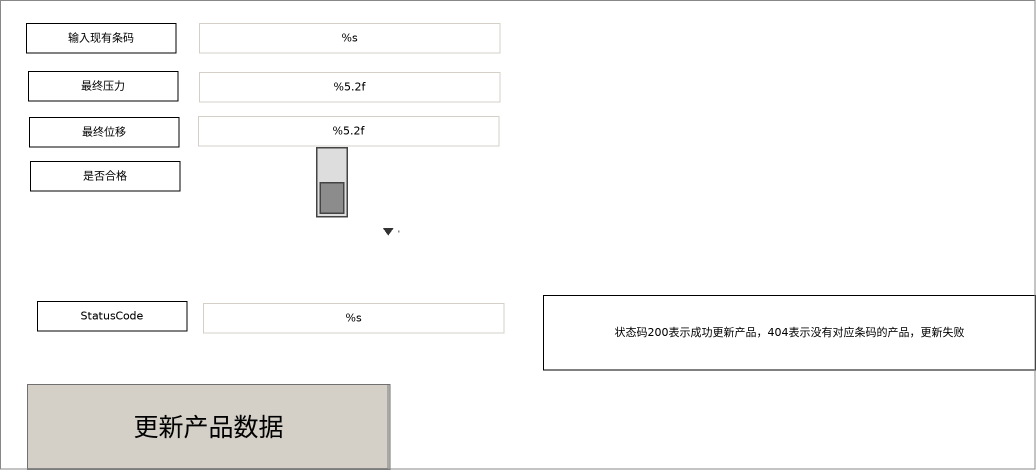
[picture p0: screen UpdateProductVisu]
VISUALIZATION UpdateProductVisu  // 1036x470
    ComboBoxInteger (398,231 1x0)
    Rectangle (26,23 150x30), "输入现有条码"
    Rectangle (28,71 150x30), "最终压力"
    Rectangle (29,117 150x30), "最终位移"
    Rectangle (30,161 150x30), "是否合格"
    Textfield (199,23 301x30), "%s", text variable: MAIN.fbUpdateProduc.product.BarCode
        OnMouseDown: write the text variable via Default
    Textfield (199,72 301x30), "%5.2f", text variable: MAIN.fbUpdateProduc.product.FinalPressure
        OnMouseDown: write the text variable via Default
    Textfield (198,116 301x30), "%5.2f", text variable: MAIN.fbUpdateProduc.product.FinalDisplacement
        OnMouseDown: write the text variable via Default
    DipSwitch (297,147 70x70), variable: MAIN.fbUpdateProduc.product.IsQualified, behaviour: TOGGLE, style: Switch-DipSwitch-Gray
    Button (27,384 363x86), "更新产品数据"
        tap MAIN.fbUpdateProduc.bSend
    Rectangle (37,301 150x30), "StatusCode"
    Textfield (203,303 301x30), "%s", text variable: MAIN.fbUpdateProduc.nStatusCode
        OnMouseDown: write the text variable via Default
    Rectangle (543,295 493x75), "状态码200表示成功更新产品，404表示没有对应条码的产品，更新失败"
END_VISUALIZATION
